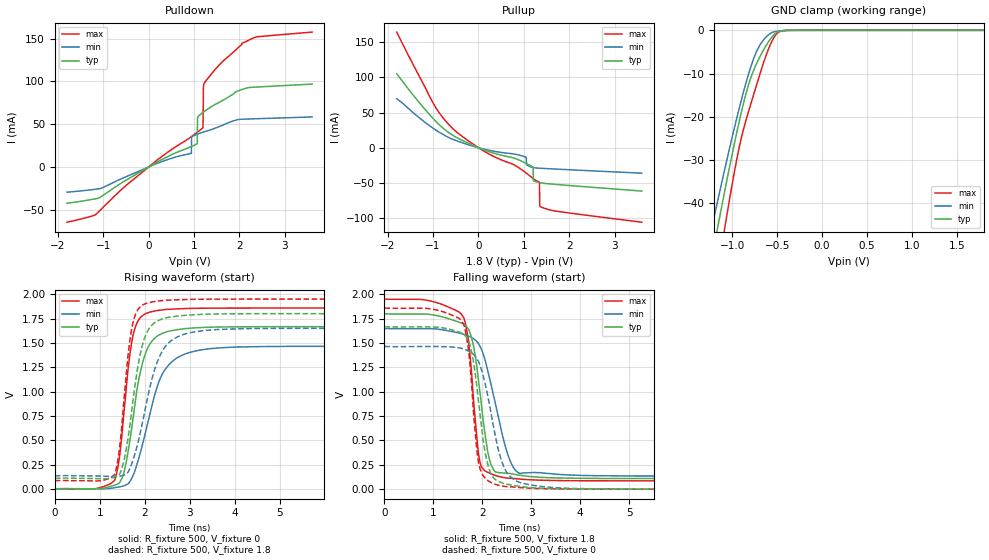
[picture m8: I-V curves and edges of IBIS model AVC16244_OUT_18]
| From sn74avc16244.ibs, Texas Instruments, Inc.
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[Model]   AVC16244_OUT_18
Model_type  3-state
Enable   Active-Low
Vref =   0
Rref =   1k
Cref =   30p
Vmeas =   0.9
| variable   typ   min   max
C_comp   4.22pF   3.35pF   5.59pF
| C_pullup   7.23pF   2.26pF   19.00pF
| C_pulldown   11.76pF   1.01pF   35.45pF
| C_tri-state   4.22pF   3.35pF   5.59pF
[Temperature Range]   40   100   -40
| Ambient temperature   25   85   -40
[Voltage range]   1.8   1.65   1.95
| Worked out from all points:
|   slope of the pulldown table from 0 to 0.27 V, typ, clamps not added: 33.5 ohm
|   slope of the pullup table from 0 to 0.27 V, typ, clamps not added: 42.5 ohm
|   GND clamp passes 1 mA (typ) near -0.53 V on its own axis
|   rising waveform, R_fixture 500, V_fixture 0: 20-80 % time 364ps typ, 529ps min, 254ps max; typ from 0 V to 1.67 V
|   falling waveform, R_fixture 500, V_fixture 1.8: 20-80 % time 268ps typ, 428ps min, 202ps max; typ from 1.8 V to 0.109 V
|   rising waveform, R_fixture 500, V_fixture 1.8: 20-80 % time 336ps typ, 490ps min, 237ps max; typ from 0.109 V to 1.8 V
|   falling waveform, R_fixture 500, V_fixture 0: 20-80 % time 265ps typ, 381ps min, 193ps max; typ from 1.67 V to 0 V
[GND Clamp]
| AVC16244_OUT_18
|   Voltage   I(typ)   I(min)   I(max)
-1.8V     -118.8mA   -103.2mA   -143.9mA
-1.215V   -51.46mA   -44.55mA   -62.92mA
-1.145V   -43.83mA   -37.92mA   -53.73mA
-1.085V   -37.42mA   -32.35mA   -46.04mA
-1.07V    -35.85mA   -30.98mA   -44.15mA
-925mV    -21.39mA   -18.32mA   -27.4mA
-825mV    -13.08mA   -10.61mA   -19.29mA
-705mV    -6.674mA   -3.925mA   -11.06mA
-575mV    -2.038mA   -727.4uA   -3.298mA
-495mV    -388.2uA   -194uA     -593.1uA
-400mV    -32.23uA   -37.99uA   -25.66uA
1.8V      937.5pA    11.16nA    32pA
[Pulldown]
| AVC16244_OUT_18
|   Voltage   I(typ)   I(min)   I(max)
-1.8V     -42.48mA   -29.53mA   -64.63mA
-1.18V    -37.33mA   -26.14mA   -56.11mA
935mV     23.8mA     15.87mA    35.26mA
950mV     24.14mA    35.36mA    35.83mA
1.065V    26.9mA     38.19mA    40.35mA
1.08V     58.17mA    38.51mA    40.96mA
1.19V     63.45mA    40.59mA    45.43mA
1.2V      63.85mA    40.76mA    59.33mA
1.205V    64.06mA    40.84mA    90.97mA
1.215V    64.46mA    40.99mA    97.19mA
2.055V    90.48mA    55.75mA    144.5mA
3.6V      96.88mA    58.46mA    157.7mA
[Pullup]
| AVC16244_OUT_18
|   Voltage   I(typ)   I(min)   I(max)
-1.8V     105.3mA    69.67mA    164.6mA
-1.02V    43.26mA    28.76mA    66.19mA
-750mV    26.33mA    17.87mA    40.3mA
-20mV     534.9uA    353.3uA    842.4uA
1.05V     -22.2mA    -13.51mA   -35.92mA
1.06V     -22.53mA   -24.37mA   -36.41mA
1.205V    -27.4mA    -28.2mA    -43.79mA
1.21V     -46.91mA   -28.26mA   -44.05mA
1.345V    -49.51mA   -29.08mA   -48.98mA
1.35V     -49.57mA   -29.1mA    -80.34mA
1.355V    -49.64mA   -29.12mA   -83.62mA
3.6V      -61.62mA   -36.17mA   -105.9mA
[Ramp]
| AVC16244_OUT_18
| variable   typ   min   max
dV/dt_r   1.00/3.73E-10   0.88/5.35E-10   1.11/2.61E-10
dV/dt_f   1.01/2.70E-10   0.91/4.35E-10   1.12/2.09E-10
R_load = 500
[Rising Waveform]
| AVC16244_OUT_18
R_fixture =   500
C_fixture =   0
L_fixture =   0
V_fixture =   0
V_fixture_min = 0
V_fixture_max = 0
|   Time   V(typ)   V(min)   V(max)
0s        20.61nV    99.68nV    745pV
1.33ns    40.71mV    15.1mV     90.6mV
1.435ns   64.2mV     23.34mV    320.7mV
1.545ns   188.7mV    36.19mV    823.4mV
1.66ns    472.4mV    71.99mV    1.349V
1.775ns   846.4mV    182mV      1.641V
2.045ns   1.427V     638.6mV    1.805V
2.465ns   1.611V     1.237V     1.843V
4.555ns   1.666V     1.462V     1.858V
40ns      1.667V     1.465V     1.858V
[Falling Waveform]
| AVC16244_OUT_18
R_fixture =   500
C_fixture =   0
L_fixture =   0
V_fixture =   1.8
V_fixture_min = 1.65
V_fixture_max = 1.95
|   Time   V(typ)   V(min)   V(max)
0s        1.8V       1.65V      1.95V
1.595ns   1.699V     1.592V     1.778V
1.725ns   1.634V     1.569V     1.488V
1.915ns   1.142V     1.498V     389.3mV
1.965ns   937.2mV    1.453V     252mV
2.175ns   256.7mV    1.08V      158.4mV
2.5ns     163mV      388.3mV    113.6mV
2.76ns    143.6mV    164mV      103.9mV
4.37ns    110.1mV    137.7mV    85.62mV
40ns      108.8mV    133.7mV    85.17mV
[Rising Waveform]
| AVC16244_OUT_18
R_fixture =   500
C_fixture =   0
L_fixture =   0
V_fixture =   1.8
V_fixture_min = 1.65
V_fixture_max = 1.95
|   Time   V(typ)   V(min)   V(max)
0s        108.8mV    133.7mV    85.17mV
1.33ns    123.1mV    130.8mV    149.8mV
1.43ns    144.5mV    133mV      386.9mV
1.535ns   288.1mV    143.8mV    907mV
1.755ns   967.1mV    323.5mV    1.738V
2ns       1.556V     800mV      1.899V
2.365ns   1.742V     1.396V     1.933V
2.915ns   1.784V     1.595V     1.945V
4.315ns   1.799V     1.647V     1.95V
40ns      1.8V       1.65V      1.95V
[Falling Waveform]
| AVC16244_OUT_18
R_fixture =   500
C_fixture =   0
L_fixture =   0
V_fixture =   0
V_fixture_min = 0
V_fixture_max = 0
|   Time   V(typ)   V(min)   V(max)
0s        1.667V     1.465V     1.858V
1.58ns    1.6V       1.443V     1.72V
1.72ns    1.521V     1.416V     1.416V
1.875ns   1.106V     1.349V     470.4mV
1.945ns   802.5mV    1.282V     222.6mV
2.155ns   183.3mV    844.1mV    74.75mV
2.33ns    80.16mV    399.2mV    40.53mV
2.5ns     49.86mV    171.4mV    25.22mV
4.415ns   807.9uV    2.817mV    338.5uV
40ns      -2.639nV   124.2nV    3.431nV
